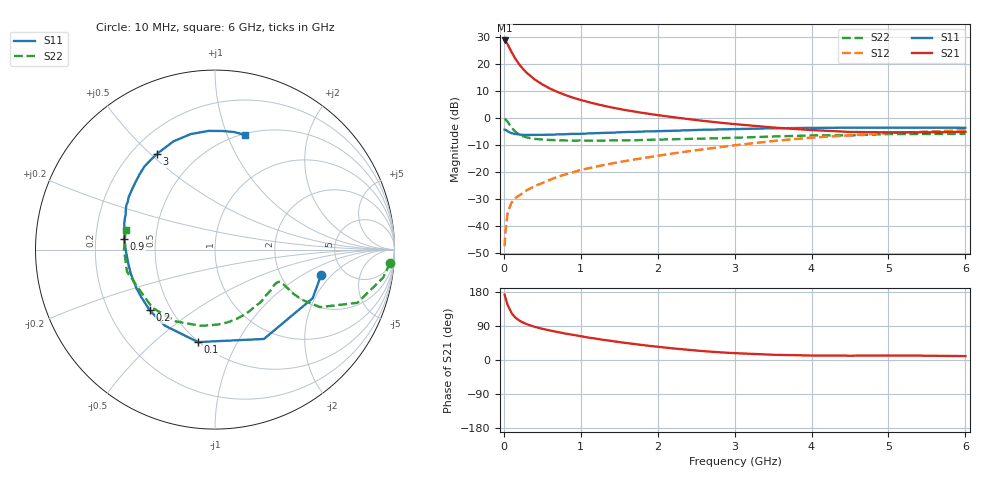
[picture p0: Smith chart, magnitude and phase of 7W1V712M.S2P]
! Infineon Technologies  Discrete & RF Semiconductors
! BFS17W
! Si NPN RF Bipolar Junction Transistor in SOT323
! VCE = 1.75 V  IC = 12 mA
! Common Emitter S-Parameters:  August  1999
# GHz  S  MA  R  50
!  f  S11  S21  S12  S22
! GHz  MAG  ANG  MAG  ANG  MAG  ANG  MAG  ANG
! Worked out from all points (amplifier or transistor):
!   36 points, 10 MHz to 6 GHz, reference 50 ohm
!   highest |S21| = 28.6 dB at 10 MHz (marker M1)
!   |S21| within 3 dB of that: start of sweep to 77.52 MHz
!   unconditionally stable (mu >= 1): 344.4 MHz to 3.081 GHz; 3.904 GHz to end of sweep
!   at 250 MHz: K = 0.89, MSG = 22.9 dB, |S12| = -27.7 dB
!   at 1.4 GHz: K = 1.25, MAG = 7.4 dB, |S12| = -16.8 dB
!   at 6 GHz: K = 1.09, MAG = -2.1 dB, |S12| = -4.5 dB
!   S11 on the Smith chart (normalised r, x): 10 MHz: 3.37, -1.52; 100 MHz: 0.50, -0.70; 200 MHz: 0.38, -0.34; 900 MHz: 0.33, +0.05; 3 GHz: 0.30, +0.52; 6 GHz: 0.51, +1.16
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0.01  0.6081 -13.5  27.05 172.6  0.0043 81.3  0.9784 -4.4
0.02  0.6078 -26.5  26.37 164.7  0.0078 80.7  0.9494 -9.5
0.05  0.5677 -61.3  22.87 144.9  0.0181 67.0  0.8468 -20.5
0.1  0.5239 -100.4  16.56 124.1  0.0274 54.1  0.667 -28.7
0.15  0.5075 -123.5  12.41 111.8  0.0334 52.1  0.557 -30.0
0.2  0.4966 -137.1  9.792 104.3  0.0372 53.2  0.4973 -29.3
0.25  0.4887 -147.1  8.023 98.7  0.0411 53.6  0.4594 -28.1
0.3  0.4878 -153.8  6.777 94.4  0.0465 55.6  0.4385 -27.3
0.4  0.4879 -163.9  5.17 87.6  0.0552 58.3  0.4114 -26.5
0.5  0.4891 -170.5  4.172 82.4  0.0631 60.8  0.4005 -26.6
0.6  0.4919 -175.4  3.49 77.8  0.0724 62.0  0.3934 -27.5
0.7  0.4975 -179.7  3.017 73.7  0.0822 63.7  0.3881 -29.1
0.9  0.5106 173.1  2.372 66.3  0.0997 64.5  0.3826 -33.1
1.1  0.519 166.7  1.967 59.3  0.1182 64.8  0.3831 -38.3
1.3  0.5316 161.0  1.683 53.0  0.1361 65.0  0.3824 -44.2
1.6  0.552 153.5  1.386 44.6  0.1622 65.2  0.3864 -53.3
2.2  0.5815 139.4  1.037 30.6  0.2218 64.5  0.4053 -73.5
3  0.624 121.2  0.772 18.1  0.3133 60.1  0.4321 -101.1
3.5  0.646 111.0  0.668 13.8  0.3761 55.2  0.4555 -118.6
4.5  0.6622 93.1  0.553 11.4  0.4784 42.6  0.4774 -152.6
5.5  0.6638 80.4  0.544 11.4  0.5621 30.6  0.507 179.9
6  0.6599 75.4  0.557 10.2  0.5949 24.9  0.5095 167.7
